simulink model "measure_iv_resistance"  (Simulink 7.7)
settings: Solver=ode8  StartTime=0.0  StopTime=5  FixedStep=0.005  RelTol=1e-300
libraries: fl_lib x5, nesl_utility x4, Memristor_lib x1

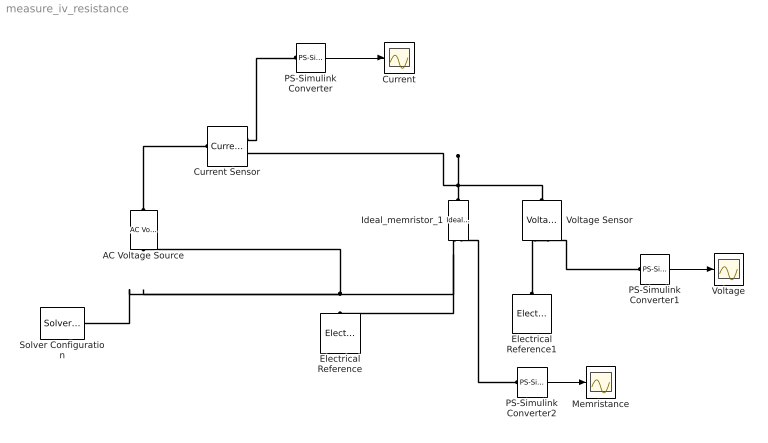
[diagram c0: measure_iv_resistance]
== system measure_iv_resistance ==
  AC Voltage Source : fl_lib/Electrical/Electrical Sources/AC Voltage Source  SystemSampleTime=-1  amp=1 V  shift=0 rad  omega=5 rad/s  i_Log=off  v_Log=off  LocalVarNames=|i|v  LocalVarDescs=|i|v  LocalVarLogging=[0 0]
  Current : Scope
  Current Sensor : fl_lib/Electrical/Electrical Sensors/Current Sensor  SystemSampleTime=-1  i1_Log=off  v1_Log=off  LocalVarNames=|i1|v1  LocalVarDescs=|i1|v1  LocalVarLogging=[0 0]
  Electrical Reference : fl_lib/Electrical/Electrical Elements/Electrical Reference  SystemSampleTime=-1  i_Log=off  LocalVarNames=|i  LocalVarDescs=|i  LocalVarLogging=0
  Electrical Reference1 : fl_lib/Electrical/Electrical Elements/Electrical Reference  SystemSampleTime=-1  i_Log=off  LocalVarNames=|i  LocalVarDescs=|i  LocalVarLogging=0
  Ideal_memristor_1 : Memristor_lib/Ideal_memristor_1  SystemSampleTime=-1  M=.005 Ohm  x0=0.4 Ohm  i_Log=off  v_Log=off  x_Log=off  LocalVarNames=|i|v|x  LocalVarDescs=|i|v|x  LocalVarLogging=[0 0 0]
  Memristance : Scope
  PS-Simulink Converter : nesl_utility/PS-Simulink Converter  SystemSampleTime=-1  PhysicalDomain=network_engine_domain  LeftPortType=input  RightPortType=output  SubClassName=ps_output  Unit=1  AffineConversion=off
  PS-Simulink Converter1 : nesl_utility/PS-Simulink Converter  SystemSampleTime=-1  PhysicalDomain=network_engine_domain  LeftPortType=input  RightPortType=output  SubClassName=ps_output  Unit=1  AffineConversion=off
  PS-Simulink Converter2 : nesl_utility/PS-Simulink Converter  SystemSampleTime=-1  PhysicalDomain=network_engine_domain  LeftPortType=input  RightPortType=output  SubClassName=ps_output  Unit=1  AffineConversion=off
  Solver Configuration : nesl_utility/Solver Configuration  SystemSampleTime=-1  PhysicalDomain=network_engine_domain  LeftPortType=input  RightPortType=generic  SubClassName=solver  Accelerate=off  Profile=off  ResidualTolerance=1e-9  MaxNonlinIter=3  MaxModeIter=2  DoFixedCost=off  UseLocalSampling=off  DoDC=off  LinearAlgebra=Sparse  LocalSolverSampleTime=.001  LocalSolverChoice=NE_BACKWARD_EULER_ADVANCER  UseLocalSolver=off
  Voltage : Scope
  Voltage Sensor : fl_lib/Electrical/Electrical Sensors/Voltage Sensor  SystemSampleTime=-1  i1_Log=off  v1_Log=off  LocalVarNames=|i1|v1  LocalVarDescs=|i1|v1  LocalVarLogging=[0 0]
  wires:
  PS-Simulink Converter/1 -> Current/1
  PS-Simulink Converter1/1 -> Voltage/1
  PS-Simulink Converter2/1 -> Memristance/1
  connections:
  Ideal_memristor_1/RConn1 -- AC Voltage Source/RConn1 -- Solver Configuration/RConn1 -- Electrical Reference/LConn1
  AC Voltage Source/LConn1 -- Current Sensor/LConn1
  Ideal_memristor_1/LConn1 -- Current Sensor/RConn2 -- Voltage Sensor/LConn1
  Current Sensor/RConn1 -- PS-Simulink Converter/LConn1
  Electrical Reference1/LConn1 -- Voltage Sensor/RConn2
  PS-Simulink Converter1/LConn1 -- Voltage Sensor/RConn1
  PS-Simulink Converter2/LConn1 -- Ideal_memristor_1/RConn2
